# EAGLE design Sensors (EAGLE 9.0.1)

## Sheet 1 of 3: Board to Board Headers
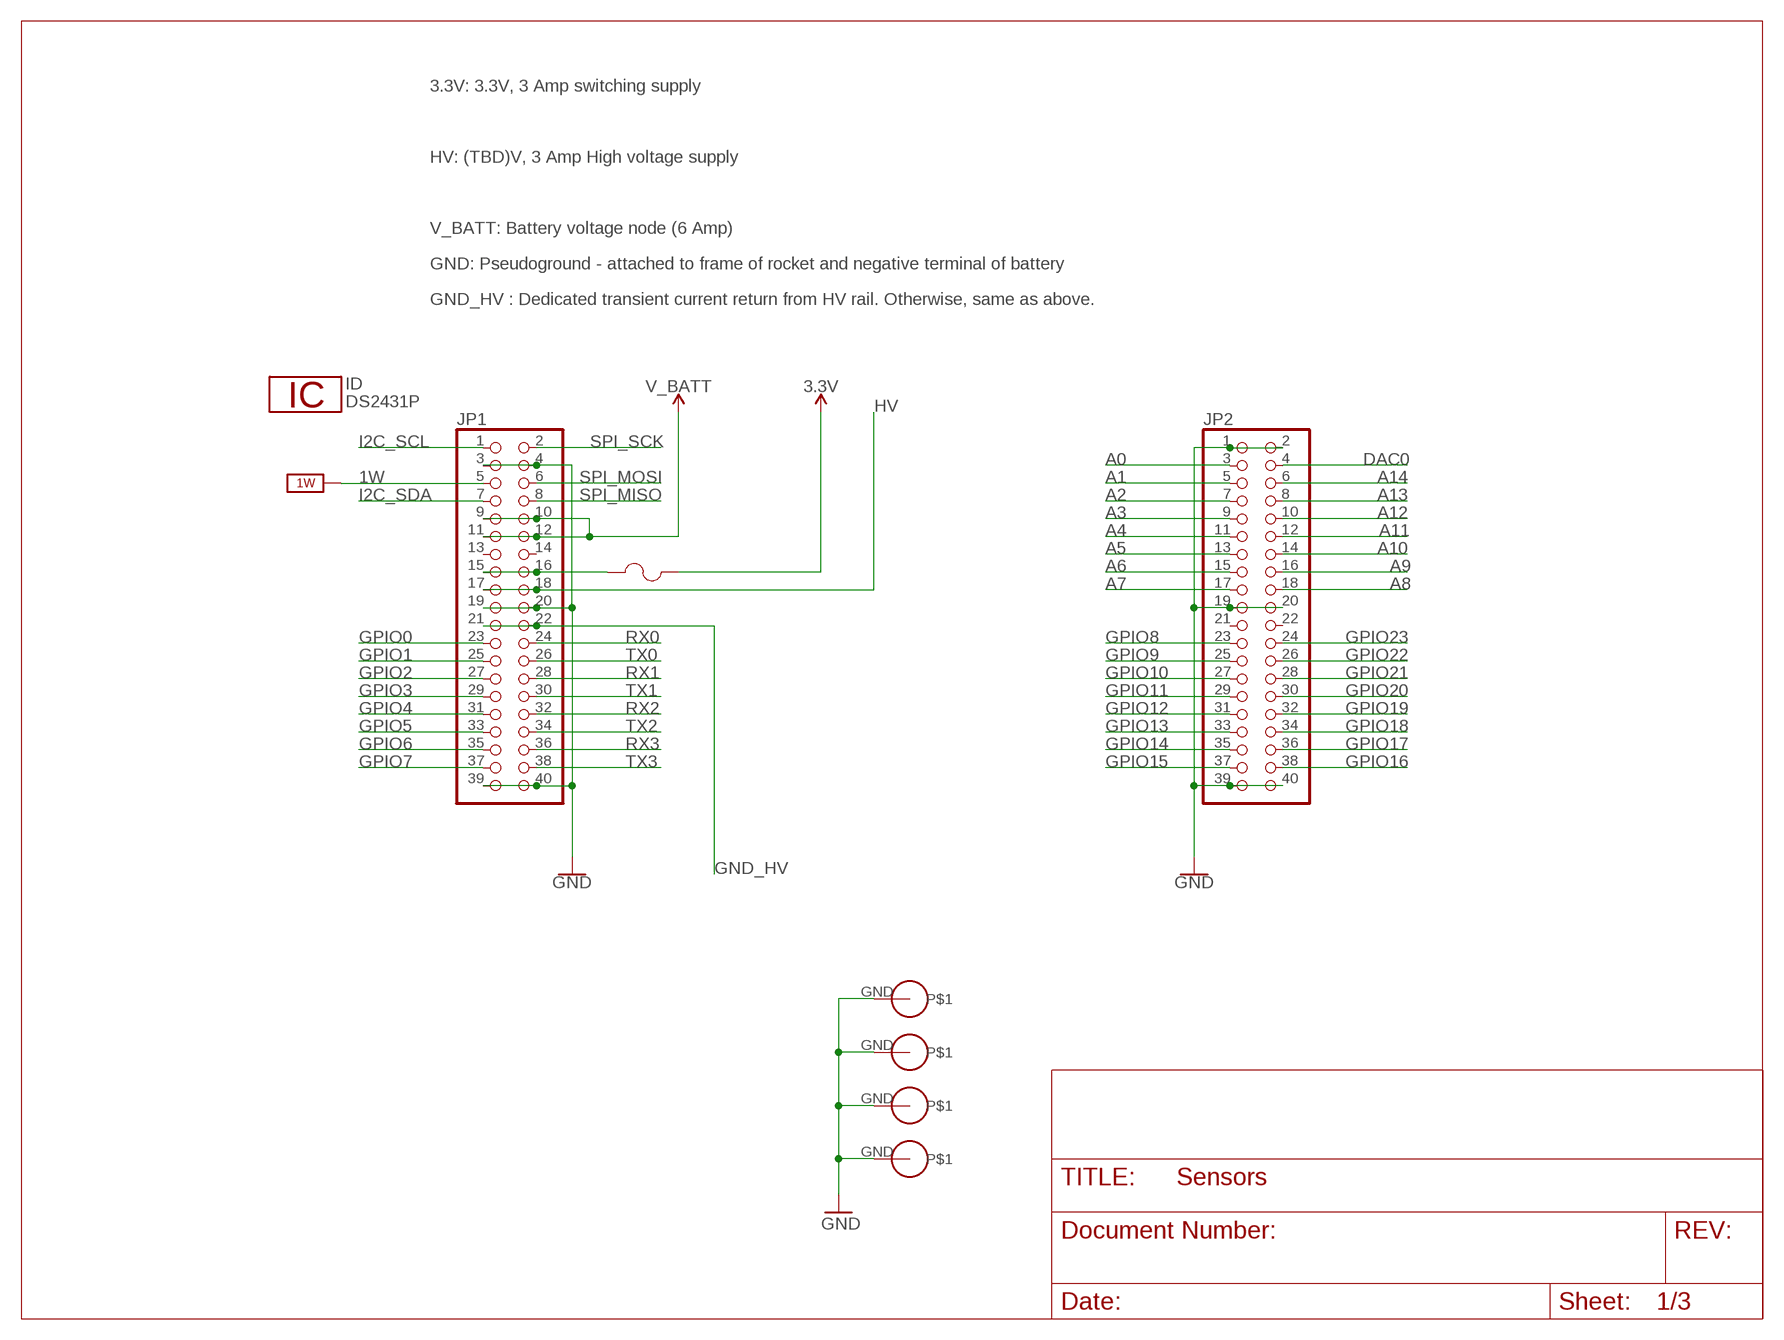
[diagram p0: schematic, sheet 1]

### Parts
F1  0603SFF150F/32-2  [FUS0603_TYCO]
ID  DS2431P  [TSOC6]
JP1  PINHD-2X20  [2X20]
JP2  PINHD-2X20  [2X20]
U$1  PS/104-MOUNTING-HOLE  [PC/104-MOUNTING-HOLE]
U$2  PS/104-MOUNTING-HOLE  [PC/104-MOUNTING-HOLE]
U$3  PS/104-MOUNTING-HOLE  [PC/104-MOUNTING-HOLE]
U$4  PS/104-MOUNTING-HOLE  [PC/104-MOUNTING-HOLE]

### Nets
1W: JP1.5 ; supply symbol labelled 1W_SUP
3.3V: F1.2 ; also sheet 2,3
A0: JP2.3
A1: JP2.5
A2: JP2.7
A3: JP2.9
A4: JP2.11
A5: JP2.13
A6: JP2.15
A7: JP2.17
A8: JP2.18
A9: JP2.16
A10: JP2.14
A11: JP2.12
A12: JP2.10
A13: JP2.8
A14: JP2.6
DAC0: JP2.4
GND: JP1.3 JP1.4 JP1.19 JP1.20 JP1.39 JP1.40 JP2.1 JP2.2 JP2.19 JP2.20 JP2.39 JP2.40 U$1.GND U$2.GND U$3.GND U$4.GND ; also sheet 2,3
GND_HV: JP1.21 JP1.22
GPIO0: JP1.23 ; also sheet 3
GPIO1: JP1.25 ; also sheet 3
GPIO2: JP1.27
GPIO3: JP1.29
GPIO4: JP1.31 ; also sheet 3
GPIO5: JP1.33 ; also sheet 3
GPIO6: JP1.35 ; also sheet 2
GPIO7: JP1.37 ; also sheet 2
GPIO8: JP2.23
GPIO9: JP2.25
GPIO10: JP2.27
GPIO11: JP2.29
GPIO12: JP2.31
GPIO13: JP2.33
GPIO14: JP2.35
GPIO15: JP2.37
GPIO16: JP2.38
GPIO17: JP2.36
GPIO18: JP2.34
GPIO19: JP2.32
GPIO20: JP2.30
GPIO21: JP2.28
GPIO22: JP2.26 ; also sheet 2
GPIO23: JP2.24 ; also sheet 2
HV: JP1.17 JP1.18
I2C_SCL: JP1.1 ; also sheet 2,3
I2C_SDA: JP1.7 ; also sheet 2,3
N$3: F1.1 JP1.15 JP1.16
RX0: JP1.24
RX1: JP1.28
RX2: JP1.32 ; also sheet 2
RX3: JP1.36 ; also sheet 2
SPI_MISO: JP1.8 ; also sheet 3
SPI_MOSI: JP1.6 ; also sheet 3
SPI_SCK: JP1.2 ; also sheet 3
TX0: JP1.26
TX1: JP1.30
TX2: JP1.34 ; also sheet 2
TX3: JP1.38 ; also sheet 2
V_BATT: JP1.9 JP1.10 JP1.11 JP1.12
Unconnected: JP1.13 JP1.14 JP2.21 JP2.22

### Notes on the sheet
- 3.3V: 3.3V, 3 Amp switching supply
- HV: (TBD)V, 3 Amp High voltage supply
- V_BATT: Battery voltage node (6 Amp)
- GND: Pseudoground - attached to frame of rocket and negative terminal of battery
- GND_HV : Dedicated transient current return from HV rail. Otherwise, same as above.

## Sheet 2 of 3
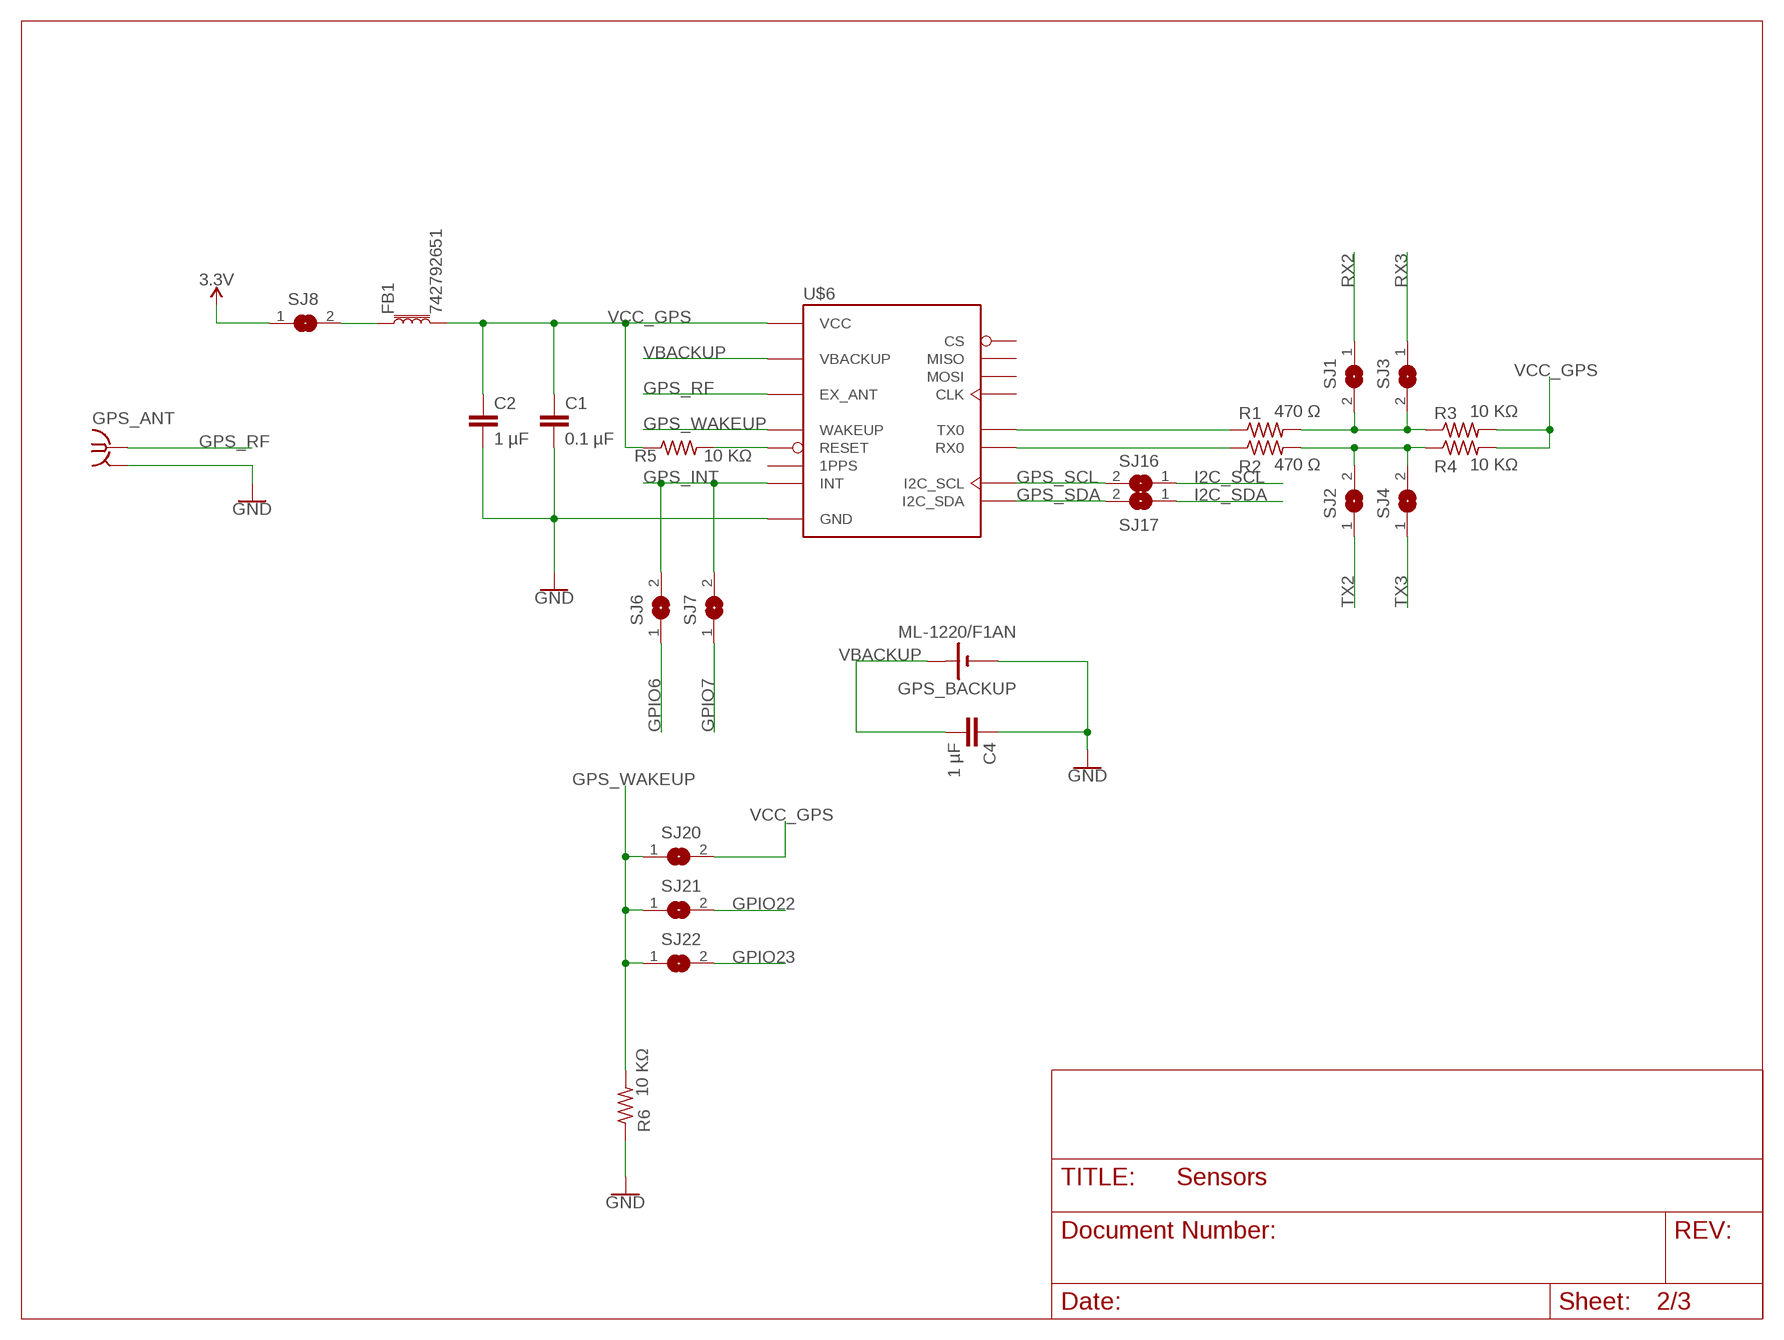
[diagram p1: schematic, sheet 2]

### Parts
C1  0.1 µF  C-EUC0805  [C0805]
C2  1 µF  C-EUC0805  [C0805]
C4  1 µF  C-EUC0805  [C0805]
FB1  742792651  FERRITE_BEAD-0603  [0603]
GPS_ANT  5MMSMA  [5MMSMA]
GPS_BACKUP  ML-1220/F1AN  [ML-1220/F1AN]
R1  470 Ω  R-US_R1206  [R1206]
R2  470 Ω  R-US_R1206  [R1206]
R3  10 KΩ  R-US_R1206  [R1206]
R4  10 KΩ  R-US_R1206  [R1206]
R5  10 KΩ  R-US_R1206  [R1206]
R6  10 KΩ  R-US_R1206  [R1206]
SJ1  SJ  [SJ]
SJ2  SJ  [SJ]
SJ3  SJ  [SJ]
SJ4  SJ  [SJ]
SJ6  SJ  [SJ]
SJ7  SJ  [SJ]
SJ8  SJ  [SJ]
SJ16  SJ  [SJ]
SJ17  SJ  [SJ]
SJ20  SJ  [SJ]
SJ21  SJ  [SJ]
SJ22  SJ  [SJ]
U$6  XA1110  [XA1110]

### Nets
3.3V: SJ8.1 ; also sheet 1,3
GND: C1.2 C2.2 C4.1 GPS_ANT.GND GPS_ANT.GND2(GND) GPS_BACKUP.NEG(N) R6.1 U$6.P$1(GND) U$6.P$3(GND) U$6.P$4(GND) U$6.P$5(GND) U$6.P$6(GND) U$6.P$9(GND) U$6.P$10(GND) U$6.P$11(GND) U$6.P$24(GND) ; also sheet 1,3
GPIO6: SJ6.1 ; also sheet 1
GPIO7: SJ7.1 ; also sheet 1
GPIO22: SJ21.2 ; also sheet 1
GPIO23: SJ22.2 ; also sheet 1
GPS_INT: SJ6.2 SJ7.2 U$6.P$16(INT)
GPS_RF: GPS_ANT.RF U$6.P$2(EX_ANT)
GPS_RX: R2.2 R4.1 SJ2.2 SJ4.2
GPS_SCL: SJ16.2 U$6.P$14(I2C_SCL)
GPS_SDA: SJ17.2 U$6.P$13(I2C_SDA)
GPS_TX: R1.2 R3.1 SJ1.2 SJ3.2
GPS_WAKEUP: R6.2 SJ20.1 SJ21.1 SJ22.1 U$6.P$12(WAKEUP)
I2C_SCL: SJ16.1 ; also sheet 1,3
I2C_SDA: SJ17.1 ; also sheet 1,3
N$1: R1.1 U$6.P$19(TX0)
N$2: R2.1 U$6.P$20(RX0)
N$4: FB1.1 SJ8.2
N$5: R5.2 U$6.P$22(RESET)
RX2: SJ1.1 ; also sheet 1
RX3: SJ3.1 ; also sheet 1
TX2: SJ2.1 ; also sheet 1
TX3: SJ4.1 ; also sheet 1
VBACKUP: C4.2 GPS_BACKUP.POS(P) U$6.P$8(VBACKUP)
VCC_GPS: C1.1 C2.1 FB1.2 R3.2 R4.2 R5.1 SJ20.2 U$6.P$7(VCC)
Unconnected: U$6.P$15(MISO) U$6.P$17(MOSI) U$6.P$18(CLK) U$6.P$21(1PPS) U$6.P$23(CS)

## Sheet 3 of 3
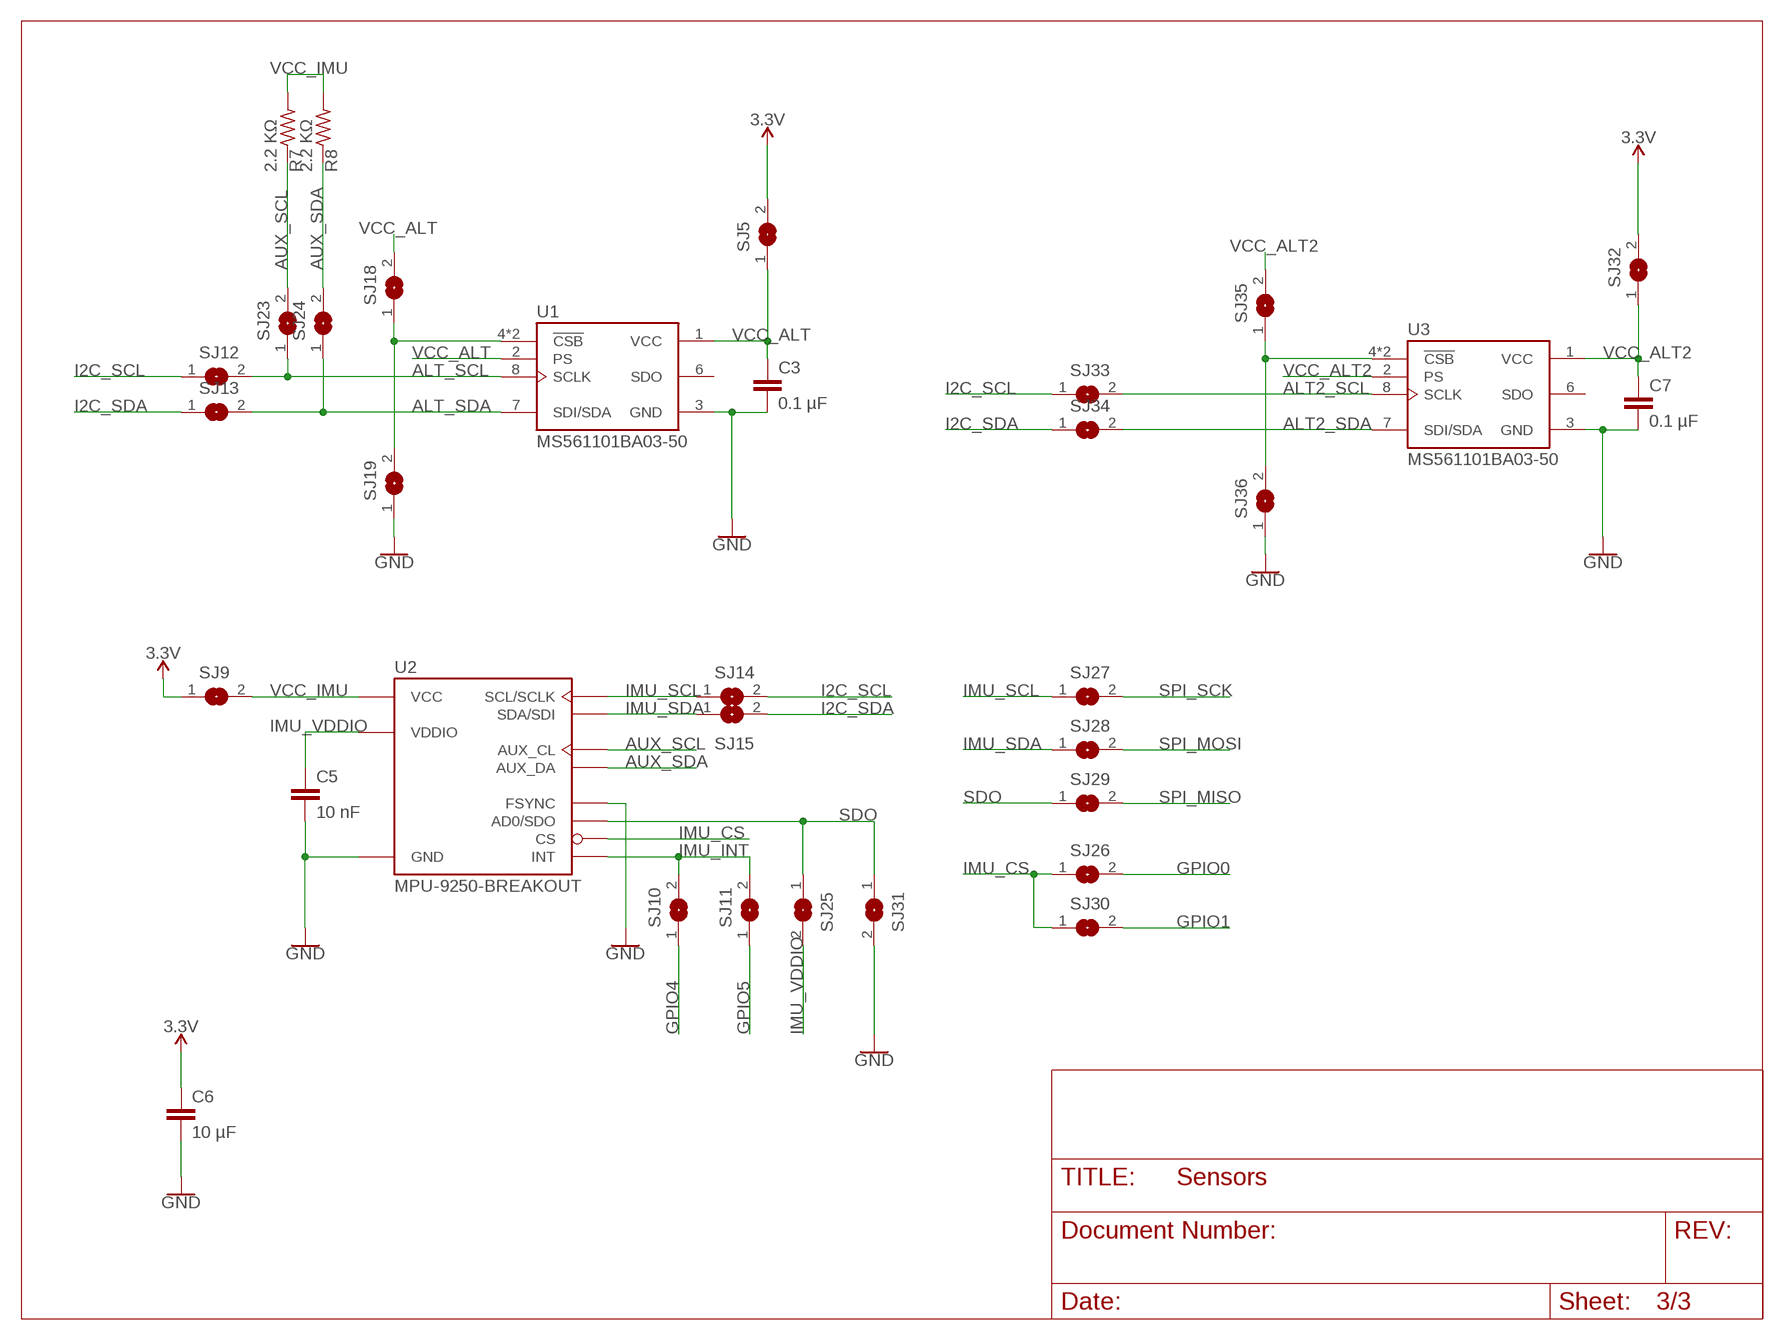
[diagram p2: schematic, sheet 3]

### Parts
C3  0.1 µF  C-EUC0805  [C0805]
C5  10 nF  C-EUC0805  [C0805]
C6  10 µF  C-EUC1206  [C1206]
C7  0.1 µF  C-EUC0805  [C0805]
R7  2.2 KΩ  R-US_R1206  [R1206]
R8  2.2 KΩ  R-US_R1206  [R1206]
SJ5  SJ  [SJ]
SJ9  SJ  [SJ]
SJ10  SJ  [SJ]
SJ11  SJ  [SJ]
SJ12  SJ  [SJ]
SJ13  SJ  [SJ]
SJ14  SJ  [SJ]
SJ15  SJ  [SJ]
SJ18  SJ  [SJ]
SJ19  SJ  [SJ]
SJ23  SJ  [SJ]
SJ24  SJ  [SJ]
SJ25  SJ  [SJ]
SJ26  SJ  [SJ]
SJ27  SJ  [SJ]
SJ28  SJ  [SJ]
SJ29  SJ  [SJ]
SJ30  SJ  [SJ]
SJ31  SJ  [SJ]
SJ32  SJ  [SJ]
SJ33  SJ  [SJ]
SJ34  SJ  [SJ]
SJ35  SJ  [SJ]
SJ36  SJ  [SJ]
U1  MS561101BA03-50  [SON125P500X300X100-8N]
U2  MPU-9250-BREAKOUT  [MPU-9250-BREAKOUT]
U3  MS561101BA03-50  [SON125P500X300X100-8N]

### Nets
3.3V: C6.1 SJ5.2 SJ9.1 SJ32.2 ; also sheet 1,2
ALT2_SCL: SJ33.2 U3.8(SCLK)
ALT2_SDA: SJ34.2 U3.7(SDI/SDA)
ALT_SCL: SJ12.2 SJ23.1 U1.8(SCLK)
ALT_SDA: SJ13.2 SJ24.1 U1.7(SDI/SDA)
AUX_SCL: R7.1 SJ23.2 U2.AUX_CL
AUX_SDA: R8.1 SJ24.2 U2.AUX_DA
GND: C3.2 C5.2 C6.2 C7.2 SJ19.1 SJ31.2 SJ36.1 U1.3(GND) U2.FSYNC U2.GND U3.3(GND) ; also sheet 1,2
GPIO0: SJ26.2 ; also sheet 1
GPIO1: SJ30.2 ; also sheet 1
GPIO4: SJ10.1 ; also sheet 1
GPIO5: SJ11.1 ; also sheet 1
I2C_SCL: SJ12.1 SJ14.2 SJ33.1 ; also sheet 1,2
I2C_SDA: SJ13.1 SJ15.2 SJ34.1 ; also sheet 1,2
IMU_CS: SJ26.1 SJ30.1 U2.NCS(CS)
IMU_INT: SJ10.2 SJ11.2 U2.INT
IMU_SCL: SJ14.1 SJ27.1 U2.SCL/SCLK
IMU_SDA: SJ15.1 SJ28.1 U2.SDA/SDI
IMU_VDDIO: C5.1 SJ25.2 U2.VDDIO
N$6: SJ18.1 SJ19.2 U1.4(!CSB) U1.5(!CSB)
N$7: SJ35.1 SJ36.2 U3.4(!CSB) U3.5(!CSB)
SDO: SJ25.1 SJ29.1 SJ31.1 U2.AD0/SDO
SPI_MISO: SJ29.2 ; also sheet 1
SPI_MOSI: SJ28.2 ; also sheet 1
SPI_SCK: SJ27.2 ; also sheet 1
VCC_ALT: C3.1 SJ5.1 SJ18.2 U1.1(VCC) U1.2(PS)
VCC_ALT2: C7.1 SJ32.1 SJ35.2 U3.1(VCC) U3.2(PS)
VCC_IMU: R7.2 R8.2 SJ9.2 U2.VDD(VCC)
Unconnected: U1.6(SDO) U3.6(SDO)

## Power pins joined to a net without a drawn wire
1W: ID.2(1W)
GND: ID.1(GND)

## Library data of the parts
C1-C7 = rcl:C-EU: CAPACITOR, European symbol; SPICEPREFIX: C
F1 = CU inSpace 2019 Parts:0603SFF150F/32-2; MANUFACTURER_PART_NUMBER: 0603SFF150F322; VENDOR: Littelfuse Inc
FB1 = SparkFun-Coils:FERRITE_BEAD: Ferrite Bead (blocks, cores, rings, chokes, etc.); PROD_ID: NDUC-07859; VALUE: 30Ω/1.8A
GPS_ANT = CU inSpace 2019 Parts:5MMSMA
GPS_BACKUP = Sensors Board:ML-1220/F1AN
ID = 1wire:DS2431: 1024-Bit EEPROM
JP1 JP2 = pinhead:PINHD-2X20: PIN HEADER
R1-R8 = rcl:R-US_: RESISTOR, American symbol; SPICEPREFIX: R
SJ1-SJ36 = jumper:SJ: SMD solder JUMPER
U1 U3 = Sensors Board:MS561101BA03-50: BAROMETRIC PRESSURE SENSOR; AVAILABILITY: Unavailable; COMMENT: MS561101BA03-50; DESCRIPTION: Barometric Pressure Sensor; EU_ROHS_COMPLIANCE: Compliant; MF: TE Connectivity; MP: MS561101BA03-50; PACKAGE: SMD-8 TE Connectivity; PRICE: None; TE_PURCHASE_URL: https://www.te.com/usa-en/product-MS561101BA03-50.html?te_bu=Cor&te_type=disp&te_campaign=seda_glo_cor-seda-global-disp-prtnr-fy19-seda-model-bom-cta_sma-317_1&elqCampaignId=32493
U2 = Sensors Board:MPU-9250-BREAKOUT
U$1-U$4 = CU inSpace 2019 Parts:PS/104-MOUNTING-HOLE: Mounting hole for PC/104 board.
U$6 = Sensors Board:XA1110

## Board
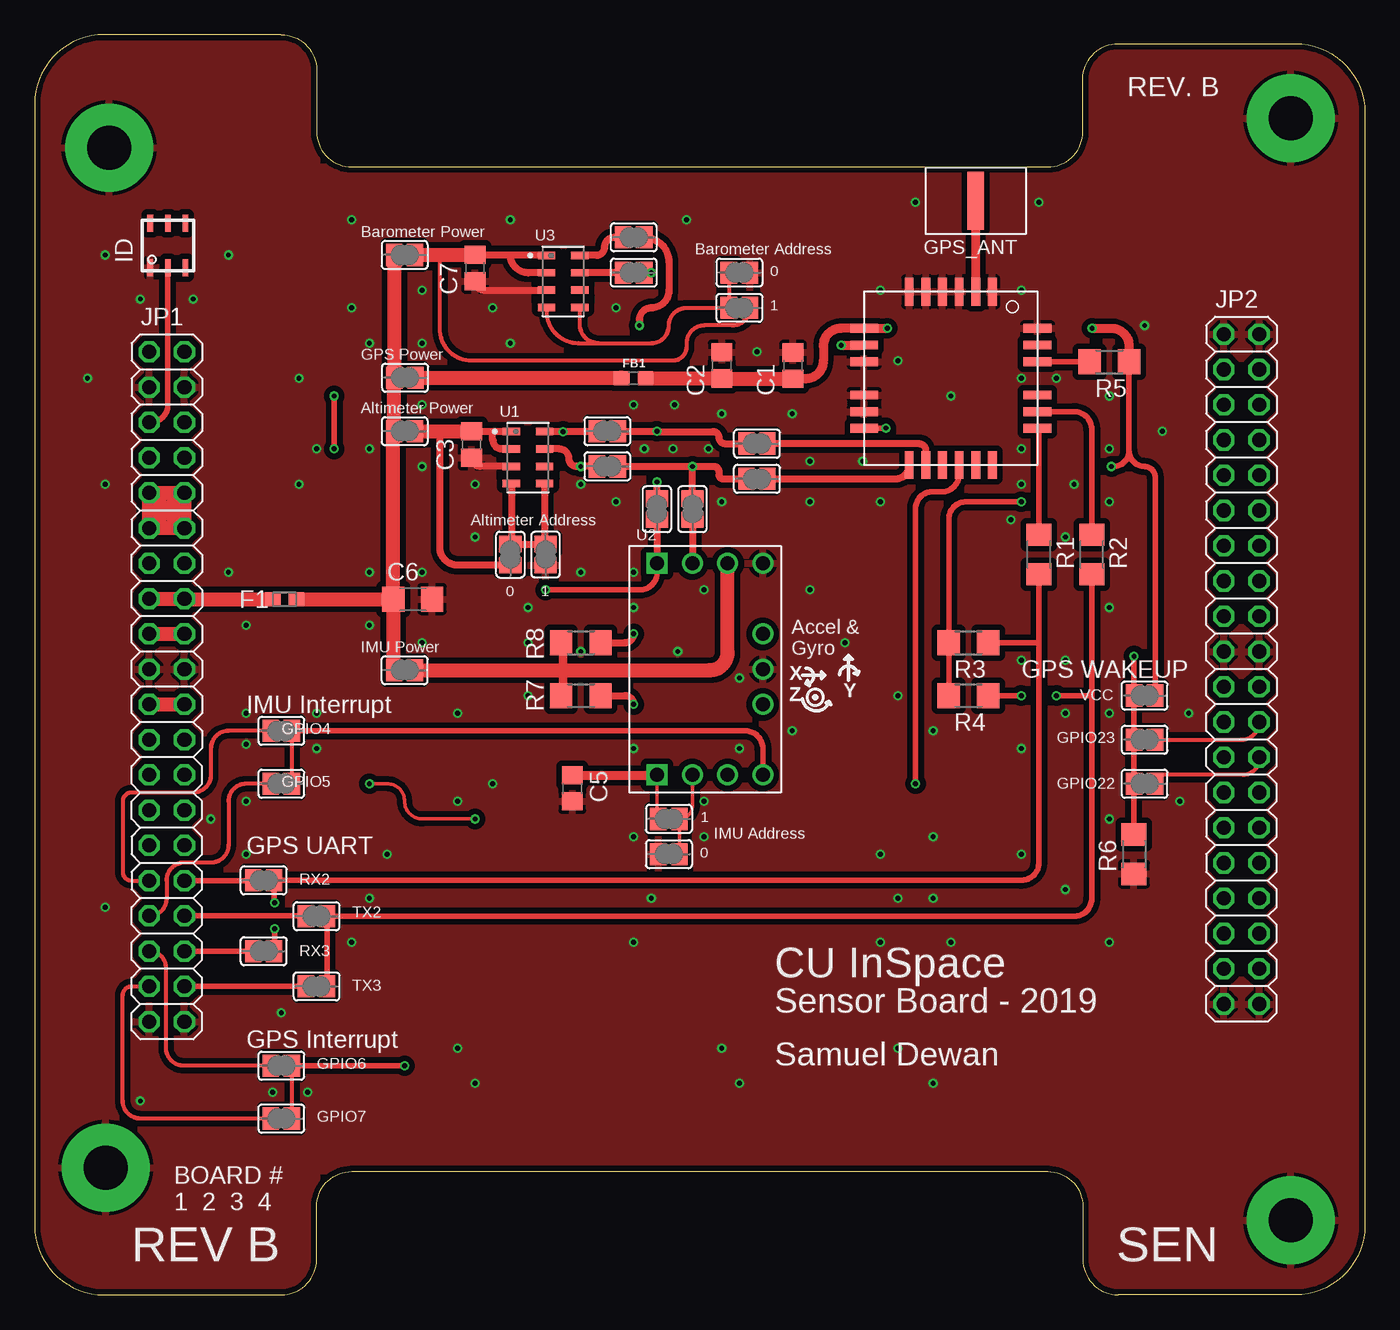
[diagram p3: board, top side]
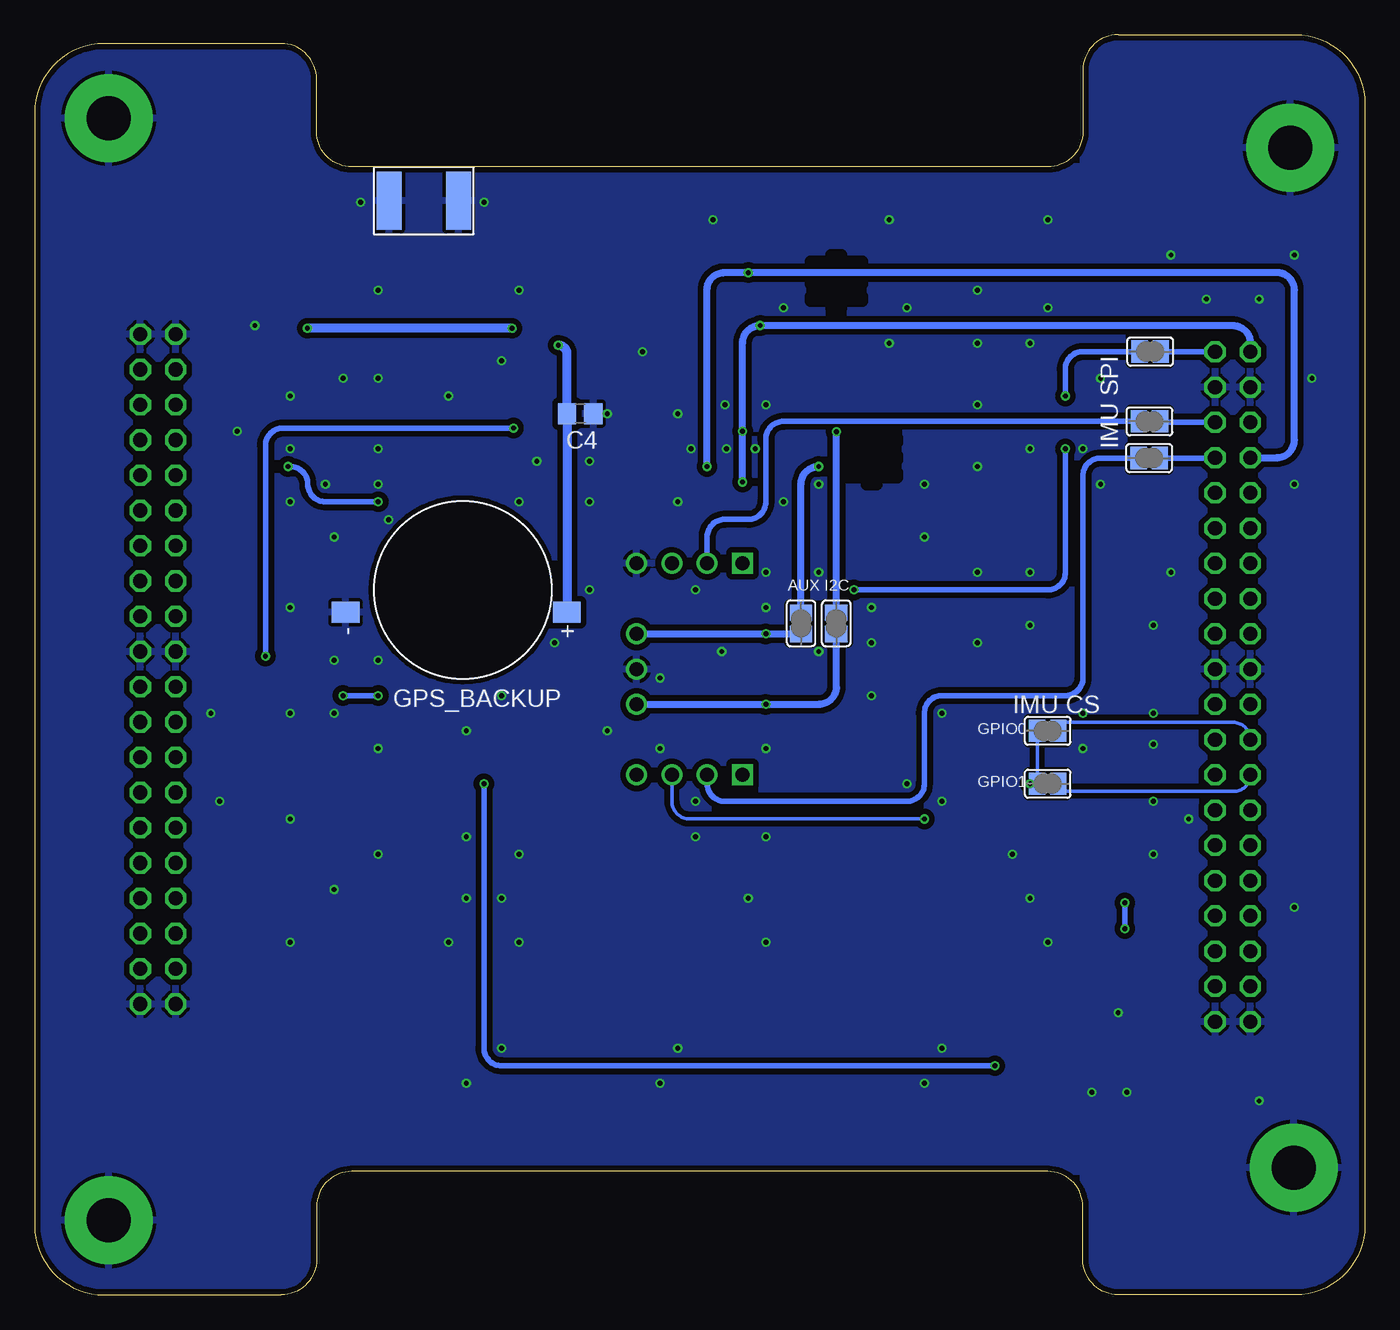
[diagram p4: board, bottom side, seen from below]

Size 95.89 x 90.81 mm. Coordinates in mm from the lower left corner, seen from the top.
Outline: 0,85.81 0,5 arc90 5,0 17.78,0 arc90 20.32,2.54 20.32,6.35 arc-90 22.86,8.89 73.03,8.89 arc-90 75.56,6.35 75.56,2.54 arc90 78.11,0 90.89,0 arc90 95.89,5 95.89,85.17 arc90 90.89,90.17 78.11,90.17 arc90 75.56,87.63 75.56,83.82 arc-90 73.03,81.28 22.86,81.28 arc-90 20.32,83.82 20.32,88.27 arc90 17.78,90.81 5,90.81 arc90 0,85.81
Copper layers (1*16): Top 0.035mm / dielectric 1.5mm / Bottom 0.035mm
Design rules "JLCPCB": minimum track width 3.5mil, minimum drill 0.2mm, track to track 5mil, track to pad 5mil, pad to pad 5mil, via to via 5mil, smd to smd 0mil, copper to edge 10mil, drill to drill 10mil, minimum pad ring 3mil, minimum via ring 6mil, stop-mask expansion 2mil, vias tented up to drill 25mil, thermal gap 10mil

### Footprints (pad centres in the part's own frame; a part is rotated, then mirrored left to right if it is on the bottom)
C0805 = smd 1.3 x 1.5: 1 -0.95,0; 2 0.95,0
C1206 = smd 1.6 x 1.8: 1 -1.4,0; 2 1.4,0
FUS0603_TYCO = smd 1.092 x 0.991: 1 -0.851,0; 2 0.851,0
0603 = smd 1.1 x 1: 1 -0.85,0; 2 0.85,0
5MMSMA = smd 1.8 x 4.2 bottom: GND 2.5,0; GND2 -2.5,0 | smd 1.2 x 4.2: RF 0,0
ML-1220/F1AN = smd 1.5 x 2: NEG -1.625,8.45; POS -1.625,-7.5
TSOC6 = smd 0.406 x 1.219: 1 -1.27,-1.6; 2 0,-1.6; 3 1.27,-1.6; 4 1.27,1.6; 5 0,1.6; 6 -1.27,1.6
2X20 = drill 1.016 octagon: 1 -24.13,-1.27; 2 -24.13,1.27; 3 -21.59,-1.27; 4 -21.59,1.27; 5 -19.05,-1.27; 6 -19.05,1.27; 7 -16.51,-1.27; 8 -16.51,1.27; 9 -13.97,-1.27; 10 -13.97,1.27; 11 -11.43,-1.27; 12 -11.43,1.27; 13 -8.89,-1.27; 14 -8.89,1.27; 15 -6.35,-1.27; 16 -6.35,1.27; 17 -3.81,-1.27; 18 -3.81,1.27; 19 -1.27,-1.27; 20 -1.27,1.27; 21 1.27,-1.27; 22 1.27,1.27; 23 3.81,-1.27; 24 3.81,1.27; 25 6.35,-1.27; 26 6.35,1.27; 27 8.89,-1.27; 28 8.89,1.27; 29 11.43,-1.27; 30 11.43,1.27; 31 13.97,-1.27; 32 13.97,1.27; 33 16.51,-1.27; 34 16.51,1.27; 35 19.05,-1.27; 36 19.05,1.27; 37 21.59,-1.27; 38 21.59,1.27; 39 24.13,-1.27; 40 24.13,1.27
R1206 = smd 1.6 x 1.803: 1 -1.422,0; 2 1.422,0
SJ = smd 1.168 x 1.6: 1 -0.762,0; 2 0.762,0
SON125P500X300X100-8N = smd 1.31 x 0.53: 1 -1.2,1.875; 2 -1.2,0.625; 3 -1.2,-0.625; 4 -1.2,-1.875; 5 1.2,-1.875; 6 1.2,-0.625; 7 1.2,0.625; 8 1.2,1.875
MPU-9250-BREAKOUT = drill 1.016: AD0/SDO -0.533,-7.62; AUX_CL 4.547,-2.54; AUX_DA 4.547,2.54; FSYNC 4.547,0; GND 4.547,7.62; INT 4.547,-7.62; NCS 2.007,-7.62; SDA/SDI -0.533,7.62; VDD 2.007,7.62 | drill 1.016 square: SCL/SCLK -3.073,7.62; VDDIO -3.073,-7.62
PC/104-MOUNTING-HOLE = drill 3.175 pad 6.35: GND 0,0
XA1110 = smd 2 x 0.635: P$1 -6.25,3; P$2 -6.25,1.8; P$3 -6.25,0.6; P$4 -6.25,-0.6; P$5 -6.25,-1.8; P$6 -6.25,-3; P$13 6.25,-3; P$14 6.25,-1.8; P$15 6.25,-0.6; P$16 6.25,0.6; P$17 6.25,1.8; P$18 6.25,3 | smd 0.635 x 2: P$7 -3.6,-6.25; P$8 -2.4,-6.25; P$9 -1.2,-6.25; P$10 1.2,-6.25; P$11 2.4,-6.25; P$12 3.6,-6.25; P$19 3.6,6.25; P$20 2.4,6.25; P$21 1.2,6.25; P$22 -1.2,6.25; P$23 -2.4,6.25; P$24 -3.6,6.25

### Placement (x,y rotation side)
C1  54.66,66.95 90 top
C2  49.53,66.98 90 top
C3  31.5,61.26 270 top
C4  56.57,63.5 180 bottom
C5  38.76,36.5 270 top
C6  27.25,50.13 0 top
C7  31.75,73.99 270 top
F1  18.02,50.13 0 top
FB1  43.18,66.04 0 top
GPS_ANT  67.84,78.84 0 top
GPS_BACKUP  65.02,50.8 90 bottom
ID  9.6,75.62 0 top
JP1  9.53,43.81 270 top
JP2  87,45.09 270 top
R1  72.39,53.34 270 top
R2  76.2,53.34 270 top
R3  67.31,46.99 180 top
R4  67.31,43.18 180 top
R5  77.47,67.23 180 top
R6  79.25,31.75 90 top
R7  39.37,43.18 180 top
R8  39.37,46.99 180 top
SJ1  16.51,29.87 0 top
SJ2  20.32,27.28 0 top
SJ3  16.51,24.77 0 top
SJ4  20.32,22.23 0 top
SJ5  26.67,62.23 180 top
SJ6  17.78,16.51 0 top
SJ7  17.78,12.7 0 top
SJ8  26.7,66.09 0 top
SJ9  26.67,45.01 0 top
SJ10  17.78,40.64 0 top
SJ11  17.78,36.83 0 top
SJ12  41.27,62.23 180 top
SJ13  41.27,59.69 180 top
SJ14  44.86,56.62 90 top
SJ15  47.42,56.62 90 top
SJ16  52.07,61.34 0 top
SJ17  52.07,58.8 0 top
SJ18  34.29,53.34 270 top
SJ19  36.83,53.34 90 top
SJ20  80.01,43.18 0 top
SJ21  80.01,36.83 0 top
SJ22  80.01,40.01 0 top
SJ23  38.1,48.39 270 bottom
SJ24  40.64,48.39 270 bottom
SJ25  45.72,34.29 180 top
SJ26  22.86,40.64 0 bottom
SJ27  15.47,67.97 0 bottom
SJ28  15.52,62.94 0 bottom
SJ29  15.54,60.3 0 bottom
SJ30  22.86,36.83 0 bottom
SJ31  45.72,31.75 180 top
SJ32  26.67,74.93 180 top
SJ33  43.18,76.2 180 top
SJ34  43.18,73.66 180 top
SJ35  50.8,71.12 0 top
SJ36  50.8,73.66 180 top
U1  35.56,60.33 0 top
U2  47.94,45.09 0 top
U3  38.1,73.03 0 top
U$1  5.36,82.65 0 top
U$2  90.55,84.79 0 top
U$3  5.13,9.17 0 top
U$4  90.55,5.36 0 top
U$6  66.04,66.04 270 top

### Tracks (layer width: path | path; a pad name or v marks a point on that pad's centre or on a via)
1W
  Top 0.406: JP1.5 8.33,62.87 arc90 9.6,64.14 ID.2
3.3V
  Top 1.016: F1.2 C6.1 | C6.1 25.85,45.06 SJ9.1 | C6.1 25.85,62.18 SJ5.2 25.91,66.06 SJ8.1 25.93,74.91 arc90 SJ32.2
ALT2_SCL
  Top 0.508: SJ33.2 41.78,76.2 arc90 41.07,75.49 arc-90 40.48,74.9 U3.8
ALT2_SDA
  Top 0.508: SJ34.2 arc-90 42.41,73.65 U3.7
ALT_SCL  (via drill 0.35)
  Top 0.508: SJ12.2 arc-90 40.48,62.2 v38.1,62.2 U1.8
  Bottom 0.508: SJ23.1 v38.1,62.2
ALT_SDA  (via drill 0.35)
  Top 0.508: SJ13.2 v39.37,59.69 39.09,59.69 arc-90 38.51,60.27 arc90 37.83,60.95 U1.7
  Bottom 0.508: v39.37,59.69 arc-90 40.64,58.42 SJ24.1
AUX_SCL  (via drill 0.35)
  Top 0.508: R7.1 42.55,43.18 arc-90 v43.18,42.55
  Bottom 0.508: U2.AUX_CL v43.18,42.55 39.37,42.55 arc-90 38.1,43.81 SJ23.2
AUX_SDA  (via drill 0.35)
  Top 0.508: R8.1 42.55,46.99 arc90 v43.18,47.62
  Bottom 0.508: U2.AUX_DA v43.18,47.62 SJ24.2
GND  (via drill 0.35)
  Top 0.508: U1.3 32.11,59.7 arc-90 C3.2 | C7.2 arc90 32.39,72.4 U3.3
  other vias: 31.75,58.42 31.75,54.61 41.91,57.15 48.26,50.8 50.8,39.37 43.18,39.37 20.32,39.37 20.32,41.91 27.94,46.99 27.94,52.07 27.94,59.69 24.13,52.07 24.13,60.96 11.43,71.75 7.62,71.75 27.94,64.14 43.18,64.14 49.53,57.15 49.53,63.5 52.07,67.94 54.61,63.5 13.97,74.93 5.08,74.93 3.81,66.04 5.08,58.42 5.08,27.94 15.24,31.75 15.24,35.56 15.24,41.91 22.86,25.4 17.78,20.32 17.14,14.61 19.68,14.61 7.62,13.97 62.23,17.78 64.77,15.24 50.8,15.24 49.53,17.78 30.48,17.78 31.75,15.24 24.13,28.57 44.45,28.57 62.23,28.57 64.77,28.57 43.18,25.4 60.96,25.4 66.04,25.4 25.4,31.75 60.96,31.75 64.77,33.02 71.12,31.75 71.12,39.37 64.77,40.64 71.12,45.72 74.93,58.42 71.12,58.42 74.3,54.61 74.3,45.72 74.3,41.91 74.3,29.21 83.19,41.91 77.47,41.91 77.47,34.29 77.47,25.4 77.47,49.53 77.47,57.15 77.47,60.96 77.47,64.77 71.12,66.04 73.66,66.04 80.01,69.85 81.28,62.23 72.39,78.74 63.5,78.74 62.23,67.31 60.96,72.39 71.12,72.39 66.04,64.77 71.12,60.96 60.96,57.15 55.88,57.15 55.88,50.8 58.42,46.99 62.23,43.18 54.61,40.64 13.97,52.07 15.24,48.26 24.13,48.26 70.38,55.85 82.55,35.56 46.13,64.14 55.88,60.07 59.69,60.07 50.8,44.45 35.56,43.18 35.56,46.99 39.37,58.42 43.18,49.53 46.35,46.35 35.56,49.53 19.05,66.04 20.32,60.96 19.05,58.42 30.48,41.91 30.48,35.56 33.02,36.83 43.18,33.02 48.26,33.02 48.26,35.56 39.37,52.07 43.18,52.07 39.37,46.35 46.02,60.96 48.56,60.96 43.94,60.96 12.7,34.29 15.24,39.67 34.29,68.58 33.02,71.12 41.91,71.12 27.94,72.39 22.86,77.47 34.29,77.47 46.99,77.47 22.86,71.12 24.13,68.58 27.94,68.58
  pour Top (isolate 0.406): 0,90.17 20.32,90.17 20.32,81.28 74.93,81.28 74.93,90.17 95.25,90.17 95.25,1.27 95.25,0 74.93,0 74.93,8.89 20.32,8.89 20.32,0 0,0
  pour Bottom (isolate 0.406): 0,90.17 20.32,90.17 20.32,81.28 74.93,81.28 74.93,90.17 95.25,90.17 95.25,0 74.93,0 74.93,8.89 20.32,8.89 20.32,0 0,0
GND_HV
  Top 1.016: JP1.21 JP1.22
GPIO0
  Bottom 0.254: JP1.23 arc-90 9.5,41.25 21.49,41.25 arc-90 SJ26.2
GPIO1
  Bottom 0.254: JP1.25 arc90 9.45,36.27 21.54,36.27 arc90 SJ30.2
GPIO4
  Top 0.305: SJ10.1 13.97,40.64 arc90 12.7,39.37 12.7,37.47 arc-90 11.43,36.2 6.99,36.2 arc90 6.35,35.56 6.35,30.48 arc90 6.99,29.84 JP1.31
GPIO5
  Top 0.305: SJ11.1 15.24,36.83 arc90 13.97,35.56 13.97,32.41 arc-90 12.7,31.14 10.77,31.14 arc90 9.5,29.87 9.5,28.55 arc-90 JP1.33
GPIO6
  Top 0.305: SJ6.1 10.74,16.51 arc-90 9.47,17.78 9.47,23.55 arc90 JP1.35
GPIO7
  Top 0.305: SJ7.1 7.62,12.7 arc-90 6.35,13.97 6.35,21.59 arc-90 6.99,22.23 JP1.37
GPIO22
  Top 0.305: JP2.26 88.27,38.63 arc-90 87.1,37.47 81.25,37.47 arc90 SJ21.2
GPIO23
  Top 0.305: SJ22.2 87,40.01 arc90 JP2.24
GPS_INT  (via drill 0.35)
  Top 0.305: SJ7.2 SJ6.2
  Top 0.406: v63.5,36.83 63.5,56.67 arc-90 64.69,57.86 65.37,57.86 arc90 66.64,59.13 U$6.P$16 | v26.67,16.51 SJ6.2
  Bottom 0.406: v63.5,36.83 63.5,17.78 arc-90 62.23,16.51 v26.67,16.51
GPS_RF
  Top 0.635: U$6.P$2 GPS_ANT.RF arc-90 GPS_ANT.RF
GPS_RX  (via drill 0.35)
  Top 0.406: SJ4.2 SJ2.2 74.93,27.28 arc90 76.2,28.55 76.2,43.18 | R2.2 76.2,43.18 | R4.1 v71.12,43.18 | v73.66,43.18 76.2,43.18
  Bottom 0.406: v71.12,43.18 v73.66,43.18
GPS_SCL
  Top 0.508: U$6.P$14 64.24,60.85 arc90 63.78,61.32 52.86,61.32 arc-90 SJ16.2
GPS_SDA
  Top 0.508: SJ17.2 62.05,58.8 arc90 U$6.P$13
GPS_TX  (via drill 0.35)
  Top 0.406: v17.3,28.25 arc-90 17.27,28.27 SJ1.2 71.12,29.87 arc90 72.39,31.14 72.39,46.99 | v17.3,26.39 17.3,24.79 arc-90 SJ3.2 | R1.2 72.39,46.99 | R3.1 72.39,46.99
  Bottom 0.406: v17.3,28.25 v17.3,26.39
GPS_WAKEUP  (via drill 0.35)
  Top 0.406: U$6.P$12 61.35,62.44 arc90 v61.37,62.46 | v79.25,46.02 SJ20.1 SJ22.1 SJ21.1 R6.2
  Bottom 0.406: v61.37,62.46 77.98,62.46 arc-90 79.25,61.19 v79.25,46.02
HV
  Top 1.016: JP1.17 JP1.18
I2C_SCL  (via drill 0.35)
  Top 0.508: SJ14.2 v44.86,58.57 | SJ12.1 v44.86,62.23 arc90 44.88,62.2 48.9,62.2 arc-90 49.33,61.77 arc90 49.76,61.34 SJ16.1 | SJ33.1 arc-90 45.72,74.42 45.72,72.39 arc-90 44.45,71.12 arc90 43.59,70.26 v43.59,69.85
  Bottom 0.508: JP1.1 8.26,68.58 arc-90 9.53,69.85 v43.59,69.85 arc-90 44.86,68.58 v44.86,62.23 v44.86,58.57
I2C_SDA  (via drill 0.35)
  Top 0.508: SJ13.1 v47.42,59.69 | SJ15.2 v47.42,59.69 | v47.42,59.69 48.97,59.69 arc-90 49.33,59.33 49.33,59.08 arc90 49.61,58.8 SJ17.1 | SJ34.1 v44.45,73.66
  Bottom 0.508: JP1.7 6.35,60.33 arc-90 5.08,61.59 5.08,72.39 arc-90 6.35,73.66 v44.45,73.66 46.18,73.66 arc-90 47.42,72.42 v47.42,59.69
IMU_CS  (via drill 0.35)
  Top 0.254: v31.75,34.29 27.94,34.29 arc-90 26.67,35.56 arc90 25.4,36.83 v24.13,36.83
  Bottom 0.254: v24.13,36.83 SJ30.1 SJ26.1 | U2.NCS 49.95,35.56 arc-90 48.68,34.29 v31.75,34.29
IMU_INT
  Top 0.305: SJ11.2 SJ10.2
  Top 0.406: U2.INT 52.49,39.37 arc90 51.22,40.64 SJ10.2
IMU_SCL  (via drill 0.35)
  Top 0.406: v21.59,64.77 v21.59,60.96 | v36.83,50.8 43.6,50.8 arc90 44.87,52.07 U2.SCL/SCLK
  Top 0.508: SJ14.1 44.86,52.72 arc90 U2.SCL/SCLK
  Bottom 0.406: SJ27.1 20.32,67.97 arc-90 21.59,66.7 v21.59,64.77 | v21.59,60.96 21.59,52.07 arc90 22.86,50.8 v36.83,50.8
IMU_SDA
  Top 0.508: SJ15.1 arc90 47.41,55.84 U2.SDA/SDI
  Bottom 0.406: SJ28.1 41.91,62.94 arc-90 43.18,61.67 43.18,57.15 arc90 44.45,55.88 46.14,55.88 arc-90 47.41,54.61 U2.SDA/SDI
IMU_VDDIO
  Top 0.254: U2.VDDIO 44.87,34.38 arc90 SJ25.2
  Top 0.635: C5.1 44.85,37.45 arc90 U2.VDDIO
N$1
  Top 0.406: U$6.P$19 arc-90 72.39,62.34 R1.1
N$2
  Top 0.406: U$6.P$20 74.93,63.64 arc-90 76.2,62.37 R2.1
N$3
  Top 1.016: JP1.15 JP1.16 10.83,50.13 F1.1
N$4
  Top 1.016: SJ8.2 42.28,66.09 FB1.1
N$5
  Top 0.406: U$6.P$22 R5.2 arc-90 R5.2
N$6
  Top 0.508: U1.5 36.76,54.17 arc90 SJ19.2 SJ18.1 arc90 34.36,54.17 U1.4
N$7
  Top 0.305: 40.64,68.58 arc-90 39.3,69.92 U3.5 | U3.4 36.9,70.87 arc90 39.19,68.58 40.64,68.58 | 40.64,68.58 44.45,68.58 arc90 45.72,69.85 arc-90 46.99,71.12 SJ35.1 SJ36.2
RX2
  Top 0.406: JP1.32 15.72,29.84 SJ1.1
RX3
  Top 0.406: JP1.36 SJ3.1
SDO
  Top 0.254: U2.AD0/SDO 47.41,35.22 arc-90 SJ25.1 SJ31.1
  Bottom 0.406: SJ29.1 19.05,60.3 arc-90 20.32,59.03 20.32,44.45 arc90 21.59,43.18 30.48,43.18 arc-90 31.75,41.91 31.75,36.83 arc90 33.02,35.56 46.14,35.56 arc90 47.41,36.83 U2.AD0/SDO
SPI_MISO
  Bottom 0.406: JP1.8 arc90 10.82,60.3 SJ29.2
SPI_MOSI
  Bottom 0.406: JP1.6 14.68,62.87 arc90 SJ28.2
SPI_SCK
  Bottom 0.406: JP1.2 14.68,67.94 arc90 SJ27.2
TX2
  Top 0.406: JP1.34 19.53,27.3 SJ2.1
TX3
  Top 0.406: JP1.38 SJ4.1
V_BATT
  Top 1.016: JP1.9 JP1.10 | JP1.10 JP1.12 | JP1.12 JP1.11 | JP1.11 JP1.9 | JP1.9 JP1.12 | JP1.11 JP1.10
VBACKUP  (via drill 0.35)
  Top 0.635: v58.14,68.43 59.78,68.43 arc90 U$6.P$8
  Bottom 0.635: v58.14,68.43 arc90 57.52,67.8 C4.2 57.52,49.18 arc90 GPS_BACKUP.POS
VCC_ALT
  Top 0.508: C3.1 33.02,62.22 | 33.02,62.22 34.34,62.22 arc-90 U1.1 | SJ18.2 30.48,52.58 arc-90 29.21,53.85 29.21,62.22 | U1.2 33.66,60.95 arc-90 33.05,61.57 arc-90 33.02,61.59 33.02,62.22
  Top 1.016: SJ5.1 arc90 27.45,62.22 29.21,62.22 C3.1
VCC_ALT2
  Top 0.305: 29.21,74.94 29.21,69.6 arc90 31.5,67.31 45.97,67.31 arc90 46.99,68.33 46.99,68.58 arc-90 48.26,69.85 50.29,69.85 arc90 SJ35.2
  Top 0.508: C7.1 34.29,74.94 | 34.29,74.94 36.86,74.94 arc-90 U3.1 | U3.2 35.58,73.65 arc-90 34.29,74.94
  Top 1.016: SJ32.1 arc-90 27.44,74.94 29.21,74.94 C7.1
VCC_GPS  (via drill 0.35)
  Top 0.406: 78.89,60.81 arc90 80.01,59.69 arc-90 80.77,58.93 SJ20.2 | 78.89,60.81 R5.1 | R4.2 R3.2 65.89,55.88 arc-90 67.16,57.15 v71.12,57.15 | v77.62,59.69 77.77,59.69 arc90 78.89,60.81
  Top 0.635: v61.47,69.65 v61.46,69.64 U$6.P$7 58.12,69.64 arc90 56.84,68.37 56.84,67.28 arc-90 55.58,66.01 54.65,66.01 | v76.22,69.65 77.62,69.65 arc-90 78.89,68.38 R5.1
  Top 1.016: C1.1 54.65,66.01 arc90 54.63,66.03 C2.1 arc90 C2.1 FB1.2
  Bottom 0.406: v71.12,57.15 74.93,57.15 arc90 76.2,58.42 arc-90 77.47,59.69 v77.62,59.69
  Bottom 0.635: v61.47,69.65 v76.22,69.65
VCC_IMU
  Top 0.61: R8.2 38.1,46.84 38.1,45.01 38.1,43.33 R7.2
  Top 1.016: SJ9.2 38.1,45.01 48.68,45.01 arc90 49.95,46.28 U2.VDD

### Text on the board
tPlace: BOARD # / 1 2 3 4 | REV B | SEN
tNames: REV. B | Barometer Power | Barometer Address | 0 | 1 | GPS Power | Altimeter Power | Altimeter Address | 0 | 1 | IMU Power | GPS WAKEUP | VCC | IMU Interrupt | GPIO4 | GPIO23 | GPIO5 | GPIO22 | 1 | IMU Address | GPS UART | 0 | RX2 | TX2 | RX3 | CU InSpace | TX3 | Sensor Board - 2019 | GPS Interrupt | Samuel Dewan | GPIO6 | GPIO7
bNames: IMU SPI | AUX I2C | IMU CS | GPIO0 | GPIO1

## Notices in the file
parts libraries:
SparkFun-PowerSymbols: Licensing: Creative Commons ShareAlike 4.0 International - https://creativecommons.org/licenses/by-sa/4.0
